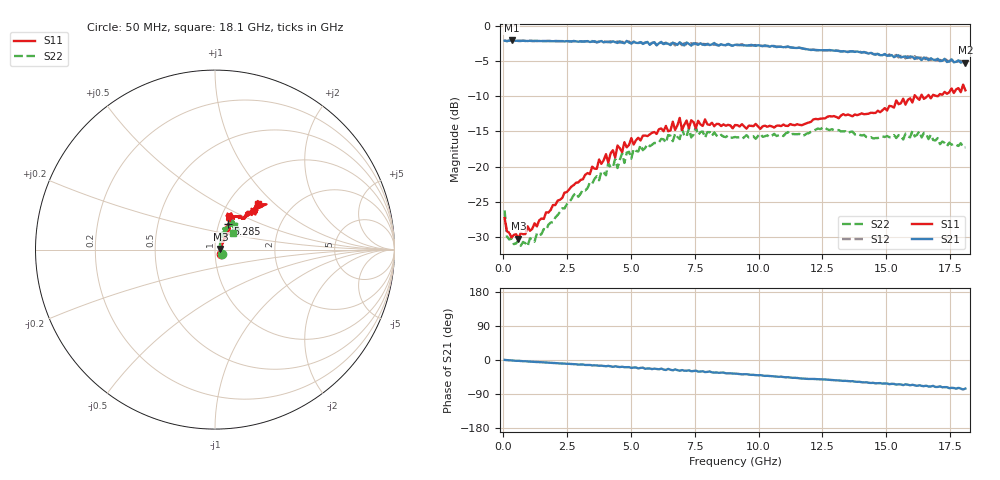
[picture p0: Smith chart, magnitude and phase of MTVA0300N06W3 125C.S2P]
! Network Analyzer HP8720D.06.14 Serial No. US36140669
!  7 Jul 2005  10:29:52
! Frequency  S11  S21  S12  S22
# HZ  S  DB R 50
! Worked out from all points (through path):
!   201 points, 50 MHz to 18.1 GHz, reference 50 ohm
!   highest |S21| = -2.09 dB at 320.8 MHz (marker M1); lowest = -5.2 dB at 18.1 GHz (marker M2)
!   group delay of S21, straight-line fit = 11.7 ps
!   lowest |S11| = -30.3 dB at 591.5 MHz (marker M3), VSWR 1.06, Z = 53.1 + j0.404 ohm
!   |S11| at or under -10 dB: start of sweep to 16.1 GHz; 16.15 GHz to 16.36 GHz (210.4 MHz wide, 1.29 % of centre); 16.42 GHz to 16.61 GHz (192.7 MHz wide, 1.17 % of centre)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
!   |S22| runs from -31.3 to -14.4 dB; largest |S21 - S12| = 0.04
!   S11 on the Smith chart (normalised r, x): 50 MHz: 1.07, -0.05; 5.285 GHz: 1.11, +0.32; 18.1 GHz: 1.37, +0.79
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5e7  -27.31 -33.1  -2.12 0.3  -2.12 0.5  -26.23 -33.2
1.4025e8  -29.19 -18.4  -2.19 -0.3  -2.18 -0.4  -29.92 -19.0
3.2075e8  -30.08 -2.9  -2.09 -1.0  -2.12 -1.0  -30.19 -5.6
5.915e8  -30.25 7.1  -2.13 -2.1  -2.17 -2.2  -30.51 8.5
1.22325e9  -28.05 26.5  -2.17 -5.0  -2.15 -4.9  -30.67 24.6
3.1185e9  -21.81 51.3  -2.25 -11.8  -2.27 -12.3  -23.29 62.6
4.021e9  -18.24 56.9  -2.29 -16.6  -2.29 -15.6  -21.24 62.8
4.11125e9  -19.44 57.4  -2.26 -15.4  -2.34 -16.7  -19.48 63.3
4.47225e9  -17.01 54.4  -2.44 -17.8  -2.24 -17.1  -20.21 68.5
4.65275e9  -17.96 55.0  -2.40 -17.6  -2.28 -19.1  -18.10 68.0
4.743e9  -16.53 58.6  -2.48 -19.1  -2.38 -18.1  -19.49 64.5
5.2845e9  -15.91 62.8  -2.45 -22.2  -2.49 -21.5  -17.87 58.9
6.09675e9  -14.69 61.5  -2.49 -24.6  -2.39 -24.3  -16.55 60.3
6.909e9  -13.09 65.8  -2.34 -28.3  -2.42 -26.6  -16.10 56.1
6.99925e9  -14.79 65.6  -2.60 -26.6  -2.76 -28.7  -14.64 56.8
7.36025e9  -13.43 61.2  -2.82 -29.6  -2.49 -28.7  -15.87 60.1
7.54075e9  -14.59 64.2  -2.60 -27.9  -2.47 -30.9  -14.42 58.7
9.075e9  -14.10 68.2  -2.70 -35.9  -2.68 -36.1  -15.80 48.6
1.21435e10  -13.31 58.6  -3.42 -49.9  -3.37 -50.1  -14.97 51.6
1.512175e10  -11.38 46.2  -4.25 -63.8  -4.08 -63.2  -15.83 48.3
1.6295e10  -10.52 41.0  -4.61 -66.6  -4.52 -69.7  -14.99 44.2
1.81e10  -9.17 46.3  -5.23 -75.4  -5.46 -76.7  -17.27 42.6
